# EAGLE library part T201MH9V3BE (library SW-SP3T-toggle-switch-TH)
Toggle Switches ON ON ON SPDT Source: Datasheet
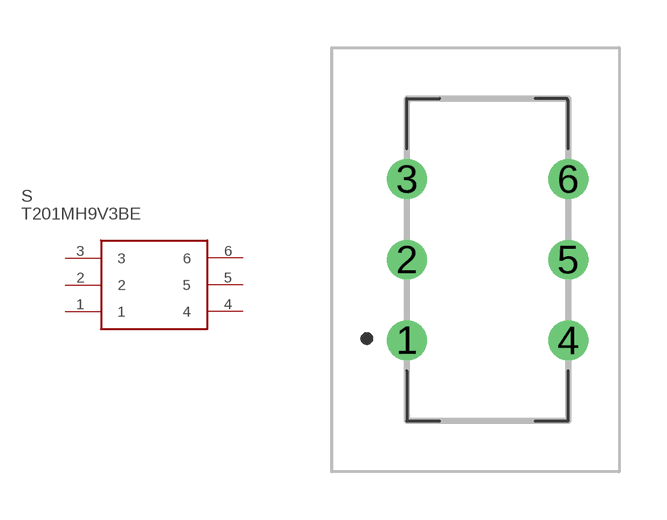
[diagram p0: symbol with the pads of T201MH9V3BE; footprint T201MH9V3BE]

Designator prefix S

## T201MH9V3BE (DESCRIPTION: Toggle Switches ON None ON DPDT 20VAC 20VDC 0.4W; HEIGHT: 20mm; MFR: C & K COMPONENTS; MPN: T211SY9CQE; VALUE: T211SY9CKE)  [T201MH9V3BE]
1  1
2  2
3  3
4  4
5  5
6  6

## Footprint T201MH9V3BE (pad centres in mm)
T211SY9CQE
drill 0.75 pad 1.2: 1 -2.54,-2.54; 2 -2.54,0; 3 -2.54,2.54; 4 2.54,-2.54; 5 2.54,0; 6 2.54,2.54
